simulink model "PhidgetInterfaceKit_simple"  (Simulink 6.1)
settings: Solver=VariableStepDiscrete  StartTime=0.0  StopTime=10  FixedStep=0.1  RelTol=1e-3
libraries: Phidgets x1, rtc x1

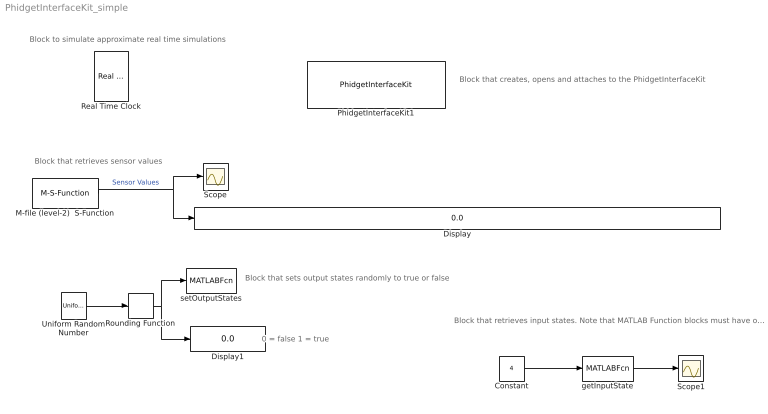
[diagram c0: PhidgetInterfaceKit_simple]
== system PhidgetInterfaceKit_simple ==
  note: 0 = false 1 = true
  note: Block that creates, opens and attaches to the PhidgetInterfaceKit
  note: Block that retrieves sensor values
  note: Block that sets output states randomly to true or false
  note: Block that retrieves input states. Note that MATLAB Function blocks must have one input block. However, the input block is never used in the getInputState M Function
  note: Block to simulate approximate real time simulations
  Constant : Constant  Value=4
  Display : Display
  Display1 : Display
  M-file (level-2)  S-Function : M-S-Function  MFile=getSensorValues
  PhidgetInterfaceKit1 : Phidgets/PhidgetInterfaceKit  serial=-1
  Real Time Clock : rtc/Real Time Clock
  Rounding Function : Rounding  Operator=round
  Scope : Scope
  Scope1 : Scope
  Uniform Random Number : UniformRandomNumber  Minimum=0  SampleTime=0
  getInputState : MATLABFcn  MATLABFcn=getInputState  OutputDimensions=8
  setOutputStates : MATLABFcn  MATLABFcn=setOutputStates  OutputDimensions=0
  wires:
  M-file (level-2)  S-Function/1 -> Scope/1, Display/1  "Sensor Values"
  Uniform Random Number/1 -> Rounding Function/1
  Rounding Function/1 -> setOutputStates/1, Display1/1
  getInputState/1 -> Scope1/1
  Constant/1 -> getInputState/1
